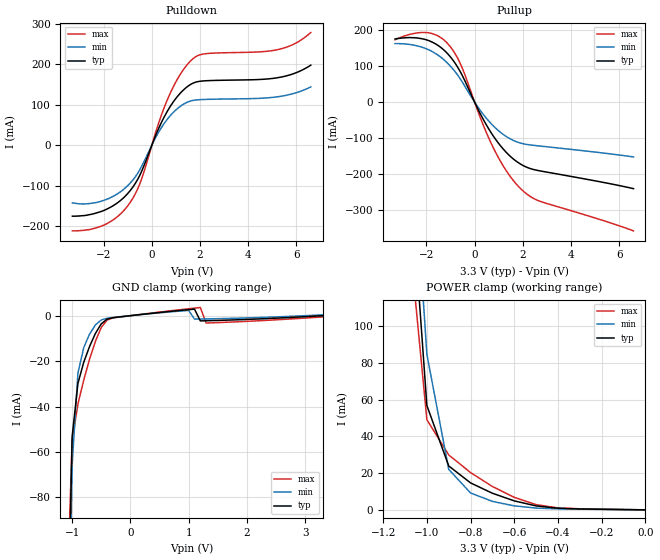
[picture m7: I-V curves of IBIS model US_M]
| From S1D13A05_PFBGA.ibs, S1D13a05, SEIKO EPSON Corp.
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[Model]   US_M
Model_type I/O
Enable Active-Low
Polarity Non-Inverting
Vinh=2.0
Vinl=0.8
C_comp   5p   4p   6p
[Temperature Range] 50   100   0
[Voltage Range]   3.3   3.0   3.6
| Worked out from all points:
|   slope of the pulldown table from 0 to 0.495 V, typ, clamps not added: 7.29 ohm
|   slope of the pullup table from 0 to 0.495 V, typ, clamps not added: 7.69 ohm
|   GND clamp passes 1 mA (typ) near -0.32 V on its own axis
|   POWER clamp passes 1 mA (typ) near -0.41 V on its own axis
[Pullup]
-3.3V     175.6mA    162.7mA    173.3mA
-2.7V     179.5mA    160.3mA    188.2mA
-2V       173.3mA    148.2mA    193.5mA
-1.5V     156.8mA    129.7mA    183.4mA
-1.1V     133.3mA    106.8mA    161.5mA
-600mV    85.25mA    65.06mA    108.2mA
300mV     -40.75mA   -29.06mA   -54.19mA
900mV     -106.4mA   -74.28mA   -143.5mA
1.5V      -152.3mA   -103.3mA   -209.1mA
2.1V      -179.7mA   -117.4mA   -252.6mA
2.8V      -192.8mA   -123.2mA   -278.5mA
6.6V      -241.3mA   -153mA     -358.9mA
[Pulldown]
-3.3V     -175.6mA   -142.6mA   -211.9mA
-1.9V     -159.1mA   -134.5mA   -195mA
-1.3V     -136.7mA   -115.1mA   -170mA
-900mV    -112.4mA   -93.87mA   -141.6mA
-500mV    -74.51mA   -60.57mA   -95.74mA
300mV     43.84mA    34.1mA     57.97mA
700mV     89.74mA    68.6mA     120.2mA
1.2V      129.9mA    96.98mA    177.2mA
1.7V      153.3mA    110.7mA    213.6mA
2.2V      159.3mA    113.3mA    226.2mA
5.3V      167.8mA    120.5mA    237.5mA
6.6V      198mA      144.2mA    278.9mA
[GND Clamp]
-3.3V     -5.515A    -4.842A    -6.448A
-1.1V     -179.1mA   -218.3mA   -136.2mA
-1V       -53.37mA   -65.82mA   -55.33mA
-900mV    -29.77mA   -25.25mA   -38.86mA
-700mV    -13.52mA   -8.093mA   -19.12mA
-500mV    -3.589mA   -1.884mA   -5.204mA
-300mV    -897.2uA   -798.3uA   -1.003mA
1V        2.654mA    2.325mA    3.045mA
1.1V      2.886mA    -1.506mA   3.324mA
1.2V      -2.295mA   -1.465mA   3.598mA
1.3V      -2.23mA    -1.42mA    -3.233mA
3.3V      4.233nA    364.4uA    -539.3uA
[POWER Clamp]
-3.3V     5.812A     5.098A     6.78A
-1.1V     222.8mA    264.6mA    172.9mA
-1V       56.72mA    84.53mA    49.02mA
-900mV    23.87mA    22.02mA    29.85mA
-800mV    14.64mA    9.157mA    20.25mA
-700mV    9.019mA    4.602mA    12.69mA
-600mV    4.872mA    2.166mA    6.787mA
-500mV    2.138mA    958.6uA    2.831mA
-400mV    869.1uA    533.4uA    1.042mA
0V        4.232nA    4.676nA    916.2pA
[Ramp]
R_load=50
dV/dt_r   1.722E+0/2.226E-9   1.479E+0/3.330E-9   1.944E+0/1.498E-9
dV/dt_f   1.738E+0/5.031E-9   1.515E+0/8.357E-9   1.958E+0/3.159E-9
